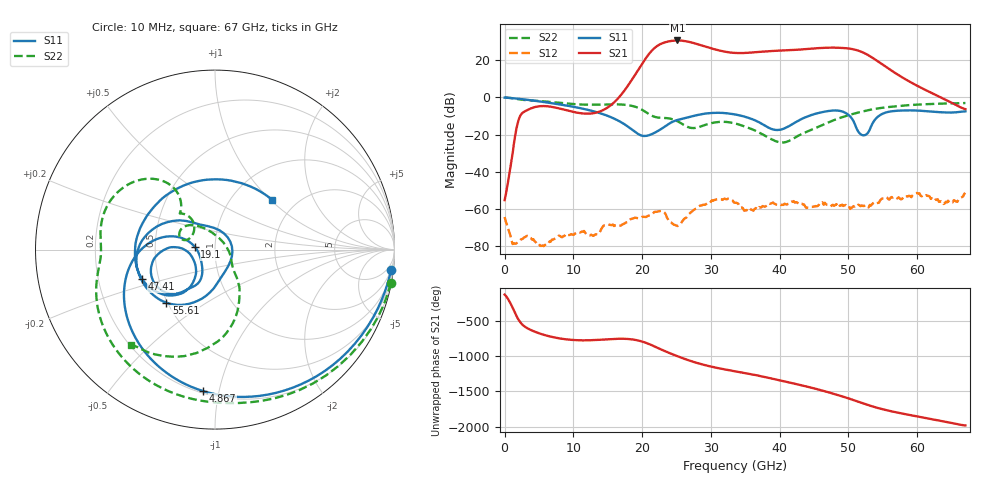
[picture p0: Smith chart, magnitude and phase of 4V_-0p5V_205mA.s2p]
! MARKI MICROWAVE INC.
! Date:  10/23/18
! Model Number:  AMM-6702CH
! Description:  2-port Small Signal S-parameter data for AMM-6702CH
! Frequency Range:  10 MHz to 67 GHz
! Port Configuration:  PORT 1: Input
!  PORT 2: Output
! Bias Condition: Vd = +4V, Vg = -0.5V
! AMM-6702CH s2p files are only valid for small signal conditions (below -5 dBm input power)
!S2P File: Measurements: Mag<S11> Ang<S11>, Mag<S21> Ang<S21>, Mag<S12> Ang<S12>, Mag<S22> Ang<S22>!row 1
# Hz S  dB  R 50
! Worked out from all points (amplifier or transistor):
!   401 points, 10 MHz to 67 GHz, reference 50 ohm
!   highest |S21| = 30.6 dB at 25.13 GHz (marker M1)
!   |S21| within 3 dB of that: 22.18 GHz to 28.94 GHz (6.765 GHz wide, 26.5 % of centre)
!   unconditionally stable (mu >= 1): start of sweep to end of sweep
!   at 11.06 GHz: K = 2434.68, MAG = -4.8 dB, |S12| = -72.6 dB
!   at 33.51 GHz: K = 18.30, MAG = 24.7 dB, |S12| = -56.7 dB
!   at 67 GHz: K = 158.95, MAG = -2.5 dB, |S12| = -51.4 dB
!   S11 on the Smith chart (normalised r, x): 10 MHz: 2, -17; 4.867 GHz: 0.21, -0.90; 19.1 GHz: 0.80, +0.02; 47.41 GHz: 0.40, -0.16; 55.61 GHz: 0.49, -0.35; 67 GHz: 1.52, +1.03
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1e7  -0.11 -6.7  -55.27 -129.3  -64.32 124.9  -0.03 -10.8
4.866775e9  -2.04 -94.9  -4.85 47.2  -78.24 -95.3  -1.88 -124.3
1.123082e10  -5.95 -165.4  -8.58 -57.9  -72.14 171.8  -3.84 -174.4
1.910215e10  -18.92 172.4  12.89 -53.7  -64.77 142.2  -5.14 134.7
2.127932e10  -19.96 -139.6  24.61 -121.3  -63.23 122.5  -9.63 125.3
2.245165e10  -17.71 -122.9  28.28 -173.4  -61.24 95.9  -10.89 132.7
2.362398e10  -14.87 -115.8  29.93 136.3  -64.74 71.7  -11.16 133.4
2.513125e10  -12.15 -121.6  30.64 77.2  -69.21 118.8  -12.80 128.0
2.6806e10  -10.60 -127.4  29.88 17.8  -62.80 129.9  -16.13 138.7
2.898318e10  -8.81 -138.5  27.59 -45.2  -57.80 107.9  -15.03 162.7
3.3505e10  -9.16 -170.3  23.92 -135.9  -56.68 53.2  -13.99 137.1
3.702198e10  -13.41 176.6  24.47 159.2  -58.96 27.0  -18.92 109.0
4.0204e10  -17.29 -144.4  25.23 91.1  -57.86 -93.9  -24.25 43.9
4.22137e10  -13.56 -124.3  25.57 46.6  -56.61 -64.5  -21.68 -12.3
4.472582e10  -9.33 -131.8  26.26 -11.9  -58.92 134.6  -17.23 -44.3
4.740542e10  -7.18 -157.8  26.76 -82.9  -58.65 139.0  -12.96 -54.7
4.874522e10  -7.25 -177.8  26.68 -121.6  -58.35 -40.2  -11.05 -60.7
5.041998e10  -10.99 145.5  26.08 -173.9  -59.49 -164.8  -9.11 -68.4
5.242968e10  -20.22 -5.4  23.62 119.0  -57.94 13.6  -7.23 -78.0
5.56117e10  -7.94 -132.5  16.01 30.6  -53.91 -154.5  -5.27 -93.6
5.594665e10  -7.65 -137.3  15.19 23.1  -54.98 -123.7  -5.14 -95.1
6.7e10  -7.48 40.8  -6.30 176.1  -51.43 -25.0  -3.03 -131.4
